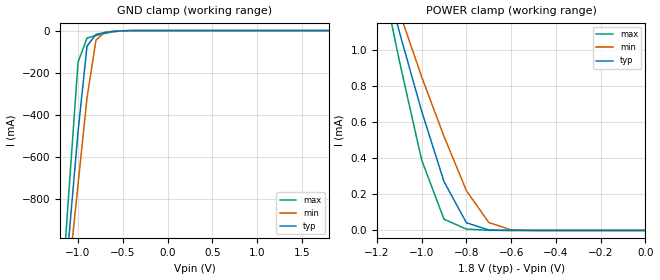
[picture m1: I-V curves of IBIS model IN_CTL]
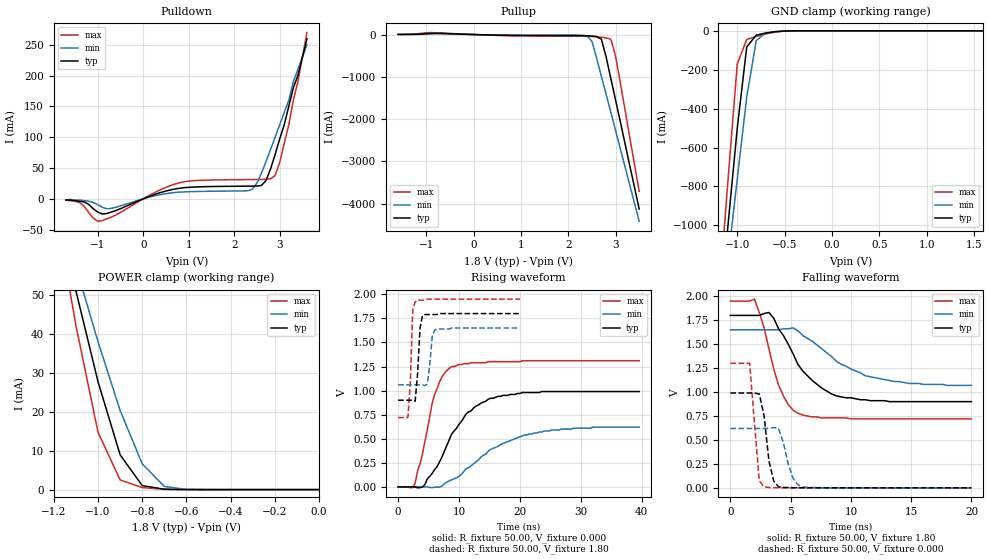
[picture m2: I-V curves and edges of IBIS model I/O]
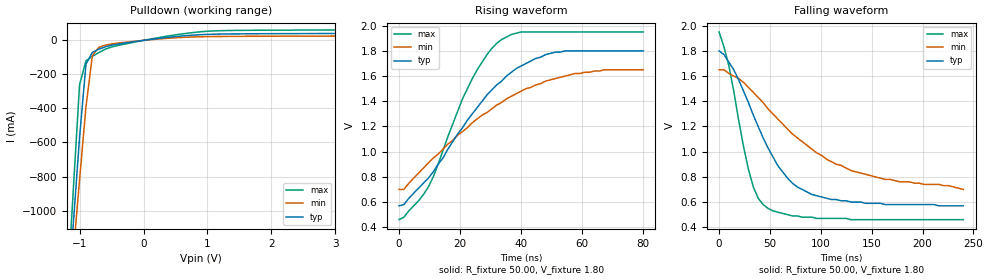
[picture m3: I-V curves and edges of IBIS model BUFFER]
| This IBIS file was created by s2ibis3 version 1.1
| North Carolina State University, ERL, 2006
[IBIS ver] 3.2
[File name] s34ms01g1_t_i_18_r2.ibs
[File Rev] 2.0
|   Rev1.0 Initial release with updated measurement
|   (X8 LEGACY/ONFI F48 98662AD 41061)
|   Rev2.0 Update 0A for 0V
[Date] 07/23/2014
[Source] Spansion IBIS team
|   Email: dl.ibisteam@spansion.com
[Notes]  Generated IBIS models from SPICE simulations.
|   VIO=1.65V - 1.95V, Temperature Range: Industrial (-40oC to +90oC).
[Disclaimer] THE MODEL LIBRARIES ARE PROVIDED AS IS.
[Copyright] (C) COPYRIGHT 2014
| SPANSION LLC
| ALL RIGHTS RESERVED.
|   Component S34MS01G1 X8 LEGACY/ONFI F48 in TSOP48 package
[Component]   S34MS01G1
[Manufacturer]   Spansion
[Package]
| variable   typ   min   max
R_pkg   216.94mOhm   199.14mOhm   240.13mOhm
L_pkg   10.66nH   7.11nH   16.8nH
C_pkg   0.87pF   0.50pF   2.33pF
[Pin]   signal_name   model_name   R_pin   L_pin   C_pin
1   NC   NC
2   NC   NC
3   NC   NC
4   NC   NC
5   NC   NC
6   NC   NC
7   R/B#   BUFFER   206.96m   8.60n   2.33p
8   RE   IN_CTL   202.33m   16.5n   0.88p
9   CE   IN_CTL   199.14m   16.8n   0.86p
10   NC   NC
11   NC   NC
12   VCC   POWER
13   VSS   GND
14   NC   NC
15   NC   NC
16   CLE   IN_CTL   202.00m   16.7n   0.87p
17   ALE   IN_CTL   205.56m   16.5n   0.89p
18   WE   IN_CTL   210.26m   12.9n   0.97p
19   WP   IN_CTL   214.96m   10.2n   1.98p
20   NC   NC
21   NC   NC
22   NC   NC
23   NC   NC
24   NC   NC
25   VSS/RFU   NC
26   NC   NC
27   NC   NC
28   NC   NC
29   IO0   I/O   240.13m   7.94n   0.52p
30   IO1   I/O   231.84m   7.85n   0.53p
31   IO2   I/O   225.21m   7.79n   0.52p
32   IO3   I/O   218.14m   7.57n   0.50p
33   NC   NC
34   VCC/RFU   NC
35   NC   NC
36   VSS   GND
37   VCC   POWER
38   NC   NC
39   VCC/RFU   NC
40   NC   NC
41   IO4   I/O   213.86m   7.52n   0.50p
42   IO5   I/O   221.30m   7.72n   0.52p
43   IO6   I/O   227.34m   7.11n   0.53p
44   IO7   I/O   234.96m   7.85n   0.51p
45   NC   NC
46   NC   NC
47   NC   NC
48   VSS/RFU   NC
| Models and submodels in the file (3): IN_CTL (Input), I/O (I/O), BUFFER (Open_drain)
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|   Model IN_CTL
[Model]   IN_CTL
Model_type   Input
Vinl =   0.36V
Vinh =   1.44V
C_comp   4.34pF   3.91pF   5.21pF
[Temperature Range]   25.00   90.00   -40.00
[Voltage Range]   1.80V   1.65V   1.95V
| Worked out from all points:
|   GND clamp passes 1 mA (typ) near -0.50 V on its own axis
|   POWER clamp passes 1 mA (typ) near -1.08 V on its own axis
[GND_clamp]
| voltage   I(typ)   I(min)   I(max)
-1.8V     -4.43A     -4.03A     -5.05A
-1.2V     -1.47A     -1.56A     -1.36A
-1.1V     -970mA     -1.14A     -750mA
-1V       -480mA     -730mA     -150mA
-900mV    -73.87mA   -320mA     -35.7mA
-800mV    -17.88mA   -45.12mA   -23.11mA
-700mV    -9.1mA     -8.55mA    -13.23mA
-600mV    -3.69mA    -2.85mA    -5.42mA
-400mV    -110uA     -120uA     -100uA
1.8V      240pA      1.3nA      110pA
[POWER_clamp]
| voltage   I(typ)   I(min)   I(max)
-1.8V     4.52mA     3.92mA     5.46mA
-1.2V     1.57mA     1.59mA     1.54mA
-1.1V     1.1mA      1.21mA     940uA
-1V       660uA      850uA      390uA
-900mV    270uA      520uA      62.17uA
-800mV    42.85uA    220uA      7.81uA
-700mV    2.54uA     43.98uA    890nA
-600mV    180nA      3.36uA     66.87nA
0V        0A         0A         0A
|   Model I/O
[Model]   I/O
Model_type   I/O
Polarity   Inverting
Enable   Active-Low
Vinl  =   0.36V
Vinh  =   1.44V
Vmeas =   0.90V
C_comp   3.48pF   3.13pF   4.18pF
[Temperature Range]   25.00   90.00   -40.00
[Voltage Range]   1.80V   1.65V   1.95V
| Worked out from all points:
|   slope of the pulldown table from 0 to 0.27 V, typ, clamps not added: 35.9 ohm
|   slope of the pullup table from 0 to 0.27 V, typ, clamps not added: 31.6 ohm
|   GND clamp passes 1 mA (typ) near -0.49 V on its own axis
|   POWER clamp passes 1 mA (typ) near -0.80 V on its own axis
|   rising waveform, R_fixture 50.00, V_fixture 0.000: 20-80 % time 5.79ns typ, 8.76ns min, 2.87ns max; typ from 0 V to 0.99 V
|   rising waveform, R_fixture 50.00, V_fixture 1.80: 20-80 % time 512ps typ, 545ps min, 455ps max; typ from 0.9 V to 1.8 V
|   falling waveform, R_fixture 50.00, V_fixture 1.80: 20-80 % time 2.97ns typ, 4.24ns min, 1.66ns max; typ from 1.8 V to 0.9 V
|   falling waveform, R_fixture 50.00, V_fixture 0.000: 20-80 % time 630ps typ, 805ps min, 510ps max; typ from 0.99 V to 0 V
[Pulldown]
| voltage   I(typ)   I(min)   I(max)
-1.7V     -2mA       -2mA       -2mA
-1.4V     -4mA       -2mA       -6mA
-1V       -21.5mA    -9.4mA     -36.5mA
-700mV    -21.55mA   -15.49mA   -29.61mA
800mV     17.17mA    10.84mA    26.12mA
2.3V      20.58mA    13.03mA    31.25mA
2.5V      20.78mA    25.63mA    31.37mA
2.7V      29.72mA    60.45mA    31.69mA
2.9V      71.92mA    100mA      37.76mA
3.2V      150mA      160mA      120mA
3.3V      180mA      190mA      160mA
3.6V      260mA      250mA      270mA
[Pullup]
| voltage   I(typ)   I(min)   I(max)
-1.6V     2.6mA      1.9mA      3.3mA
-900mV    30.55mA    14.19mA    46.85mA
700mV     -18.21mA   -11.31mA   -27.49mA
2.1V      -24.45mA   -14.19mA   -41.16mA
2.4V      -29.59mA   -34.69mA   -42.55mA
2.5V      -36.59mA   -160mA     -45.69mA
2.6V      -47.63mA   -560mA     -53.7mA
2.7V      -110mA     -990mA     -65.37mA
2.8V      -530mA     -1.41A     -79.35mA
2.9V      -1.04A     -1.84A     -110mA
3V        -1.55A     -2.27A     -510mA
3.5V      -4.13A     -4.42A     -3.71A
[GND_clamp]
| voltage   I(typ)   I(min)   I(max)
-1.6V     -3.59A     -3.33A     -3.99A
-1.2V     -1.52A     -1.61A     -1.42A
-1.1V     -1.01A     -1.19A     -780mA
-1V       -500mA     -760mA     -170mA
-900mV    -82.68mA   -340mA     -44.8mA
-800mV    -22.28mA   -50.64mA   -28.91mA
-700mV    -11.42mA   -10.58mA   -16.3mA
-600mV    -4.6mA     -3.62mA    -6.52mA
-400mV    -130uA     -150uA     -120uA
1.6V      290pA      1.71nA     140pA
[POWER_clamp]
| voltage   I(typ)   I(min)   I(max)
-1.8V     240mA      210mA      290mA
-1.2V     76.17mA    77.46mA    74.6mA
-1.1V     51.04mA    57.29mA    42.14mA
-1V       27.7mA     37.97mA    14.73mA
-900mV    8.94mA     20.33mA    2.46mA
-800mV    1.03mA     6.62mA     520uA
-700mV    97.74uA    810uA      68.2uA
-600mV    10.52uA    59.01uA    5.35uA
0V        0A         0A         0A
[Ramp]
| variable   typ   min   max
dV/dt_r   0.58/5.46n   0.31/6.36n   0.78/2.81n
dV/dt_f   0.54/2.91n   0.35/4.33n   0.74/1.55n
R_load = 50.00
[Rising Waveform]
R_fixture = 50.00
V_fixture = 0.000
V_fixture_min = 0.000
V_fixture_max = 0.000
| time   V(typ)   V(min)   V(max)
0s        0V         0V         0V
2.8ns     -26uV      220nV      37.73mV
4ns       -2.35mV    79.58uV    340mV
6ns       180mV      -2.61mV    960mV
7.2ns     310mV      8.53mV     1.14V
8.8ns     550mV      74.68mV    1.25V
11.2ns    760mV      190mV      1.28V
16.4ns    940mV      420mV      1.3V
24ns      990mV      580mV      1.31V
39.6ns    990mV      620mV      1.31V
[Rising Waveform]
R_fixture = 50.00
V_fixture = 1.80
V_fixture_min = 1.65
V_fixture_max = 1.95
| time   V(typ)   V(min)   V(max)
0s        900mV      1.06V      720mV
1.6ns     900mV      1.06V      720mV
2ns       900mV      1.06V      1.08V
2.4ns     900mV      1.06V      1.84V
2.8ns     890mV      1.06V      1.92V
3.6ns     1.65V      1.06V      1.94V
4ns       1.78V      1.06V      1.94V
4.8ns     1.79V      1.07V      1.95V
6ns       1.79V      1.63V      1.95V
20ns      1.8V       1.65V      1.95V
[Falling Waveform]
R_fixture = 50.00
V_fixture = 1.80
V_fixture_min = 1.65
V_fixture_max = 1.95
| time   V(typ)   V(min)   V(max)
0s        1.8V       1.65V      1.95V
2ns       1.8V       1.65V      1.97V
2.8ns     1.82V      1.65V      1.67V
3.2ns     1.83V      1.65V      1.45V
4ns       1.66V      1.65V      1.07V
4.8ns     1.5V       1.66V      870mV
5.6ns     1.29V      1.64V      780mV
8.4ns     980mV      1.37V      730mV
11.2ns    920mV      1.17V      720mV
20ns      900mV      1.07V      720mV
[Falling Waveform]
R_fixture = 50.00
V_fixture = 0.000
V_fixture_min = 0.000
V_fixture_max = 0.000
| time   V(typ)   V(min)   V(max)
0s        990mV      620mV      1.3V
1.6ns     990mV      620mV      1.3V
2.4ns     980mV      620mV      72.85mV
2.8ns     750mV      620mV      12.43mV
3.2ns     280mV      620mV      3.88mV
3.6ns     71.09mV    630mV      1.96mV
4ns       10.62mV    620mV      1.11mV
5.2ns     1.94mV     99.79mV    380uV
6ns       760uV      8.29mV     190uV
20ns      35.13uV    13.85uV    10.73uV
|   Model BUFFER
[Model]   BUFFER
Model_type   Open_drain
Polarity   Non-Inverting
Enable   Active-Low
Vmeas =   0.9000V
Rref =   2.0000k
Vref =   1.8000V
C_comp   3.92pF   3.53pF   4.70pF
[Temperature Range]   25.00   90.00   -40.00
[Voltage Range]   1.80V   1.65V   1.95V
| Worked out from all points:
|   slope of the pulldown table from 0 to 0.27 V, typ, clamps not added: 20.7 ohm
|   rising waveform, R_fixture 50.00, V_fixture 1.80: 20-80 % time 22.8ns typ, 29.6ns min, 15.3ns max; typ from 0.57 V to 1.8 V
|   falling waveform, R_fixture 50.00, V_fixture 1.80: 20-80 % time 44.7ns typ, 85.2ns min, 22ns max; typ from 1.8 V to 0.57 V
[Pulldown]
| voltage   I(typ)   I(min)   I(max)
-1.7V     -4.29A     -3.92A     -4.86A
-1.2V     -1.62A     -1.7A      -1.54A
-1.1V     -1.09A     -1.26A     -890mA
-1V       -570mA     -820mA     -260mA
-900mV    -140mA     -390mA     -120mA
-800mV    -70.59mA   -90.34mA   -94.24mA
-700mV    -51.91mA   -41.16mA   -71.52mA
-400mV    -21.65mA   -15.79mA   -29.77mA
300mV     14.37mA    9.95mA     20.49mA
900mV     33.57mA    21.29mA    50.74mA
1.5V      38.33mA    23.73mA    58.75mA
3.6V      40.97mA    25.68mA    61.9mA
[Ramp]
| variable   typ   min   max
dV/dt_r   0.36/11.11n   0.26/11.19n   0.55/9.56n
dV/dt_f   0.15/11.48n   50.40m/10.06n   0.44/11.38n
R_load = 50.00
[Rising Waveform]
R_fixture = 50.00
V_fixture = 1.80
V_fixture_min = 1.65
V_fixture_max = 1.95
| time   V(typ)   V(min)   V(max)
0s        570mV      700mV      460mV
1.6ns     580mV      700mV      480mV
9.6ns     790mV      910mV      720mV
20.8ns    1.19V      1.16V      1.42V
24ns      1.3V       1.23V      1.58V
28.8ns    1.45V      1.31V      1.77V
33.6ns    1.56V      1.39V      1.89V
40ns      1.68V      1.48V      1.95V
51.2ns    1.79V      1.58V      1.95V
80ns      1.8V       1.65V      1.95V
[Falling Waveform]
R_fixture = 50.00
V_fixture = 1.80
V_fixture_min = 1.65
V_fixture_max = 1.95
| time   V(typ)   V(min)   V(max)
0s        1.8V       1.65V      1.95V
9.6ns     1.71V      1.62V      1.68V
28.8ns    1.39V      1.51V      860mV
33.6ns    1.29V      1.47V      720mV
38.4ns    1.2V       1.43V      630mV
48ns      1.03V      1.34V      550mV
67.2ns    790mV      1.18V      500mV
91.2ns    660mV      1.02V      480mV
129.6ns   600mV      850mV      460mV
240ns     570mV      700mV      460mV
